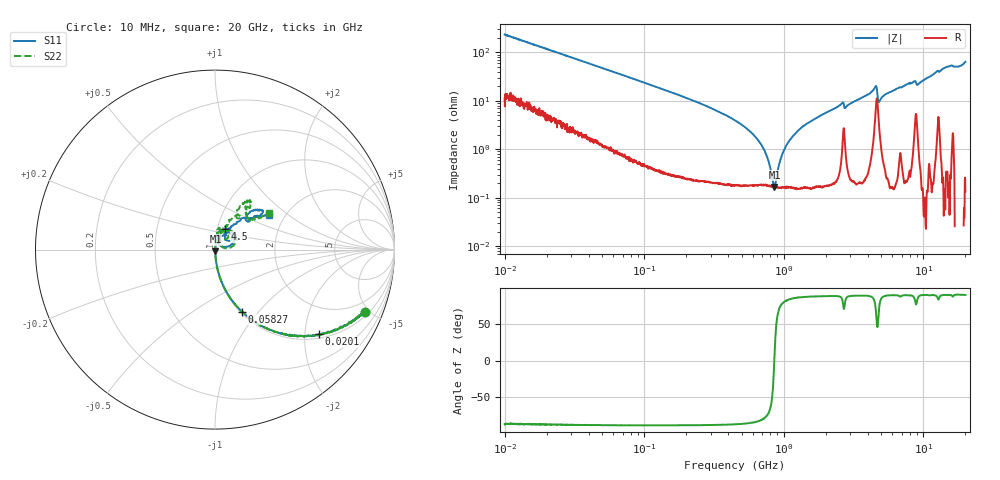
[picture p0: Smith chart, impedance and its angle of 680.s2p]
!Keysight Technologies,P5008B,MY61100088,A.16.20.02
!Date: Friday, August 30, 2024 14:27:39
!Correction: S11(C  2-Port  )
!S21(C  2-Port  )
!S12(C  2-Port  )
!S22(C  2-Port  )
!S2P File: Measurements: S11, S21, S12, S22:Log Frequency Sweep
# Hz S  MA  R 50
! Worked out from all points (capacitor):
!   1601 points, 10 MHz to 20 GHz, reference 50 ohm
!   read as one part in series: C = 68.1 pF near 10.39 MHz
!   lowest |Z| = 167 mohm at 857.4 MHz (marker M1)
!   series resonance near 855.2 MHz, so ESL is about 510 pH
!   S11 on the Smith chart (normalised r, x): 10 MHz: 1.21, -4.67; 20.1 MHz: 1.10, -2.36; 58.27 MHz: 1.02, -0.82; 4.5 GHz: 1.09, +0.25; 20 GHz: 1.66, +0.73
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1e7  0.9046 -22.7  0.3865 64.6  0.3865 64.6  0.9042 -22.7
2.010398e7  0.7474 -39.2  0.6322 48.3  0.6319 48.3  0.7472 -39.2
3.555162e7  0.5477 -55.1  0.8202 33.1  0.8199 33.1  0.5478 -55.1
5.826749e7  0.3756 -66.7  0.9185 22.0  0.9182 22.0  0.3756 -66.8
1.263918e8  0.185 -78.3  0.9795 10.5  0.9791 10.5  0.185 -78.6
4.472136e8  0.04449 -84.7  0.9975 2.0  0.9969 2.0  0.04435 -86.7
6.793157e8  0.02053 -83.7  0.998 0.3  0.9977 0.3  0.02057 -85.6
8.573649e8  0.009539 -73.8  0.9983 -0.5  0.9981 -0.5  0.009063 -88.1
9.383512e8  0.005343 -62.3  0.9985 -0.9  0.9981 -0.9  0.004574 -85.1
1.026987e9  0.002751 0.7  0.9986 -1.2  0.9981 -1.2  0.0005078 26.3
1.108091e9  0.005591 46.4  0.9986 -1.5  0.9982 -1.6  0.00418 93.0
1.184294e9  0.008563 60.4  0.9986 -1.8  0.9982 -1.8  0.007595 93.9
1.589917e9  0.02243 80.6  0.9985 -3.2  0.9979 -3.2  0.02204 85.0
2.581161e9  0.05586 77.9  0.9933 -6.6  0.9929 -6.6  0.05492 76.5
2.824976e9  0.04458 80.5  0.9949 -6.3  0.9945 -6.3  0.04405 73.2
4.4999e9  0.128 64.3  0.9565 -13.6  0.956 -13.6  0.1293 55.1
4.924959e9  0.04058 67.8  0.9859 -9.8  0.9856 -9.9  0.04453 50.9
5.652411e9  0.06751 74.4  0.9972 -13.1  0.9969 -13.1  0.07016 73.9
7.697294e9  0.1166 58.9  0.9945 -19.1  0.9939 -19.2  0.1139 78.1
9.264046e9  0.08588 47.5  0.9917 -21.6  0.9914 -21.8  0.07975 73.5
1.407205e10  0.3053 45.3  0.9643 -36.8  0.964 -37.0  0.3008 58.3
2e10  0.3576 32.6  0.9372 -56.4  0.937 -56.7  0.3617 33.9
